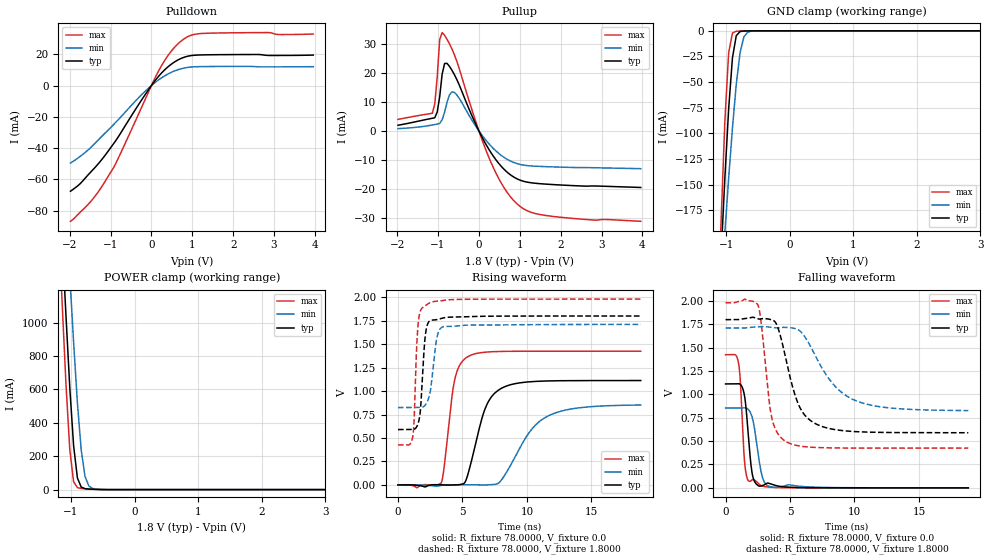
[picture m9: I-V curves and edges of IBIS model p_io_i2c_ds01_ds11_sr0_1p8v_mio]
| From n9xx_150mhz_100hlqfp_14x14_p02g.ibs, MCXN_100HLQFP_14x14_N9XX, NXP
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[Model] p_io_i2c_ds01_ds11_sr0_1p8v_mio
|   Model p_io_i2c_ds01_ds11_sr0_1p8v_mio
| This model was characterised for following simulation conditions:
| External (pad) voltage:
|   - Typ: 1.8V,   - Min: 1.71V,   - Max: 1.98V
| Library cells for typ/min/max conditions are connected as defined below:
|  pad - External Pad
|  ipp_do_lv - Core Input
|  ipp_obe_lv - Output Buffer Enable
|  IOGC - NC
|  REFH3V3 - REFH3V3
|  REFL3V3 - REFL3V3
|  ZI - NC
|  abut_ncal_vddio[1] - vssio vddio vddio
|  abut_ncal_vddio[2] - vddio vddio vssio
|  abut_ncal_vddio[3] - vddio
|  abut_ncal_vddio[4] - vssio vddio vddio
|  abut_ncal_vddio[5] - vddio vddio vssio
|  abut_ncal_vddio[6] - vddio
|  abut_pcal_vddio[1] - vssio
|  abut_pcal_vddio[2] - vddio vssio vddio
|  abut_pcal_vddio[3] - vssio
|  abut_pcal_vddio[4] - vssio
|  abut_pcal_vddio[5] - vddio vssio vddio
|  abut_pcal_vddio[6] - vssio
|  ipp_do_1p8v - ipp_do_1p8v
|  ipp_dse_lv[0] - vdd_lv
|  ipp_dse_lv[1] - vdd_lv
|  ipp_eftd_lv - NC
|  ipp_ina_mux_vddio - NC
|  ipp_ina_mux_vddio[0] - NC
|  ipp_ina_mux_vddio[1] - NC
|  ipp_ina_r0_vddio - NC
|  ipp_ina_r0a_vddio - NC
|  ipp_ina_r0b_vddio - NC
|  ipp_ina_r0c_vddio - NC
|  ipp_ina_r0d_vddio - NC
|  ipp_ina_r0e_vddio - NC
|  ipp_ina_r0f_vddio - NC
|  ipp_ina_r300_vddio - NC
|  ipp_ina_r300a_vddio - NC
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Model_type I/O
Polarity   Non-Inverting
Enable   Active-High
Vinl =   0.5400V
Vinh =   1.2600V
Vmeas =  0.9000V
Cref =   30.0000pF
Rref =   1.0000M
Vref =   1.8000V
C_comp   1.4328pF   1.3910pF   1.4871pF
|C_comp_pullup   0.6294pF   0.6726pF   0.5891pF
|C_comp_pulldown   0.7023pF   0.7084pF   0.7047pF
[Model Spec]
| variable   typ   min   max
Vinh   1.2600V   1.1970V   1.3860V
Vinl   0.5400V   0.5130V   0.5940V
[Temperature Range]   25.0000   0.1250k   -40.0000
[Voltage Range]   1.8000V   1.7100V   1.9800V
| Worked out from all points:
|   slope of the pulldown table from 0 to 0.27 V, typ, clamps not added: 31.3 ohm
|   slope of the pullup table from 0 to 0.27 V, typ, clamps not added: 38.8 ohm
|   GND clamp passes 1 mA (typ) near -0.78 V on its own axis
|   POWER clamp passes 1 mA (typ) near -0.58 V on its own axis
|   rising waveform, R_fixture 78.0000, V_fixture 0.0: 20-80 % time 1.38ns typ, 2.45ns min, 770ps max; typ from 0 V to 1.11 V
|   rising waveform, R_fixture 78.0000, V_fixture 1.8000: 20-80 % time 332ps typ, 460ps min, 269ps max; typ from 0.59 V to 1.8 V
|   falling waveform, R_fixture 78.0000, V_fixture 0.0: 20-80 % time 430ps typ, 576ps min, 323ps max; typ from 1.11 V to 0 V
|   falling waveform, R_fixture 78.0000, V_fixture 1.8000: 20-80 % time 1.49ns typ, 2.66ns min, 764ps max; typ from 1.8 V to 0.59 V
[Pulldown]
|Voltage   I(typ)   I(min)   I(max)
-1.98V    -67.59mA   -49.58mA   -86.84mA
-1.74V    -62.7mA    -45.23mA   -80.98mA
-1.44V    -54.1mA    -38.51mA   -72.8mA
-960mV    -38.41mA   -25.86mA   -54.05mA
-780mV    -31.57mA   -20.97mA   -44.79mA
-240mV    -9.218mA   -5.869mA   -13.93mA
180mV     6.058mA    3.748mA    9.583mA
420mV     12.31mA    7.625mA    19.75mA
720mV     17.31mA    10.72mA    28.38mA
960mV     19.16mA    11.86mA    32.11mA
1.26V     19.65mA    12.17mA    33.39mA
3.96V     19.52mA    12.12mA    33.02mA
[Pullup]
|Voltage   I(typ)   I(min)   I(max)
-1.98V    1.974mA    801.8uA    4.007mA
-1.14V    4.389mA    2.051mA    6.122mA
-1.08V    4.553mA    2.206mA    9.344mA
-1.02V    6.58mA     2.365mA    18.71mA
-960mV    11.81mA    2.599mA    31.64mA
-900mV    19.63mA    3.875mA    34.08mA
-780mV    23.4mA     9.952mA    31.75mA
-600mV    19.5mA     13.32mA    26.39mA
240mV     -6.288mA   -4.377mA   -9.06mA
900mV     -16.36mA   -11.18mA   -24.83mA
1.62V     -18.41mA   -12.37mA   -29.26mA
3.96V     -19.59mA   -13.08mA   -31.31mA
[GND_clamp]
|Voltage   I(typ)   I(min)   I(max)
-1.98V    -1.586A    -1.229A    -2.1A
-1.08V    -221.4mA   -253.6mA   -188.5mA
-1.02V    -144.6mA   -197.7mA   -89.32mA
-960mV    -76.59mA   -144.3mA   -21.58mA
-900mV    -26.43mA   -94.89mA   -2.183mA
-840mV    -4.754mA   -52.29mA   -428.7uA
-780mV    -708.9uA   -21.31mA   -240uA
-720mV    -194.5uA   -5.864mA   -159.9uA
-660mV    -97.62uA   -1.274mA   -100.6uA
-600mV    -55.49uA   -286.4uA   -56.47uA
-420mV    -4.265uA   -10.7uA    -2.74uA
3.96V     0A         0A         0A
[POWER_clamp]
|Voltage   I(typ)   I(min)   I(max)
-1.98V    7.929A     7.752A     8.366A
-1.2V     1.949A     2.483A     1.628A
-1.14V    1.495A     2.081A     1.12A
-1.08V    1.044A     1.68A      633.7mA
-1.02V    613.2mA    1.282A     240.4mA
-960mV    264mA      886.2mA    47.43mA
-900mV    69.94mA    519.6mA    11.58mA
-840mV    15.1mA     237.3mA    7.049mA
-780mV    5.589mA    78.54mA    5.099mA
-720mV    3.316mA    21.56mA    3.521mA
-660mV    2.102mA    6.487mA    2.205mA
3.96V     0A         0A         0A
[Ramp]
| variable   typ   min   max
dV/dt_r  0.6672/1.3789n   0.5108/2.4538n   0.8548/0.7698n
dV/dt_f  0.7261/1.4903n   0.5299/2.6602n   0.9329/0.7645n
R_load = 78.0000
[Rising Waveform]
R_fixture= 78.0000
V_fixture= 0.0
V_fixture_min= 0.0
V_fixture_max= 0.0
|time   V(typ)   V(min)   V(max)
0s        293.7pV    104.7nV    10.7pV
3.353ns   1.031mV    -6.04mV    21.16mV
4.376ns   -1.535mV   1.282mV    1.105V
5.137ns   17.27mV    557.5uV    1.338V
5.494ns   146.9mV    -583.6uV   1.373V
6.747ns   808.2mV    -626.3uV   1.414V
8.004ns   1.028V     48.68mV    1.423V
10.24ns   1.099V     569.7mV    1.425V
11.58ns   1.108V     730.4mV    1.425V
18.83ns   1.112V     851.3mV    1.425V
[Rising Waveform]
R_fixture= 78.0000
V_fixture= 1.8000
V_fixture_min= 1.7100
V_fixture_max= 1.9800
|time   V(typ)   V(min)   V(max)
0s        589.7mV    824.3mV    425.2mV
1.157ns   589.4mV    824.3mV    523.8mV
1.45ns    619.4mV    824.2mV    1.477V
1.595ns   670.1mV    824mV      1.755V
1.752ns   815.1mV    824.3mV    1.86V
2.081ns   1.54V      845.3mV    1.906V
2.334ns   1.726V     906.5mV    1.931V
3.011ns   1.762V     1.565V     1.958V
3.481ns   1.779V     1.685V     1.966V
18.83ns   1.8V       1.71V      1.98V
[Falling Waveform]
R_fixture= 78.0000
V_fixture= 0.0
V_fixture_min= 0.0
V_fixture_max= 0.0
|time   V(typ)   V(min)   V(max)
0s        1.112V     854.3mV    1.425V
1.009ns   1.114V     854.3mV    1.335V
1.149ns   1.107V     854.9mV    1.146V
1.475ns   984.1mV    857.1mV    283.1mV
1.807ns   499.6mV    832.8mV    72.72mV
2.032ns   184.7mV    770.7mV    82.48mV
2.236ns   71.88mV    644.9mV    85.14mV
2.816ns   22.89mV    138.9mV    21.34mV
3.346ns   49.69mV    17.66mV    8.379mV
18.83ns   2.136uV    25.33uV    153.9nV
[Falling Waveform]
R_fixture= 78.0000
V_fixture= 1.8000
V_fixture_min= 1.7100
V_fixture_max= 1.9800
|time   V(typ)   V(min)   V(max)
0s        1.8V       1.71V      1.98V
2.53ns    1.808V     1.723V     1.952V
2.759ns   1.809V     1.726V     1.776V
3.574ns   1.797V     1.716V     758.8mV
4.062ns   1.715V     1.712V     579.5mV
4.664ns   1.389V     1.717V     497.3mV
5.76ns    861.8mV    1.681V     447.4mV
7.329ns   664.5mV    1.319V     430.3mV
10.43ns   599.5mV    915.9mV    425.6mV
18.83ns   589.9mV    826.8mV    425.2mV
